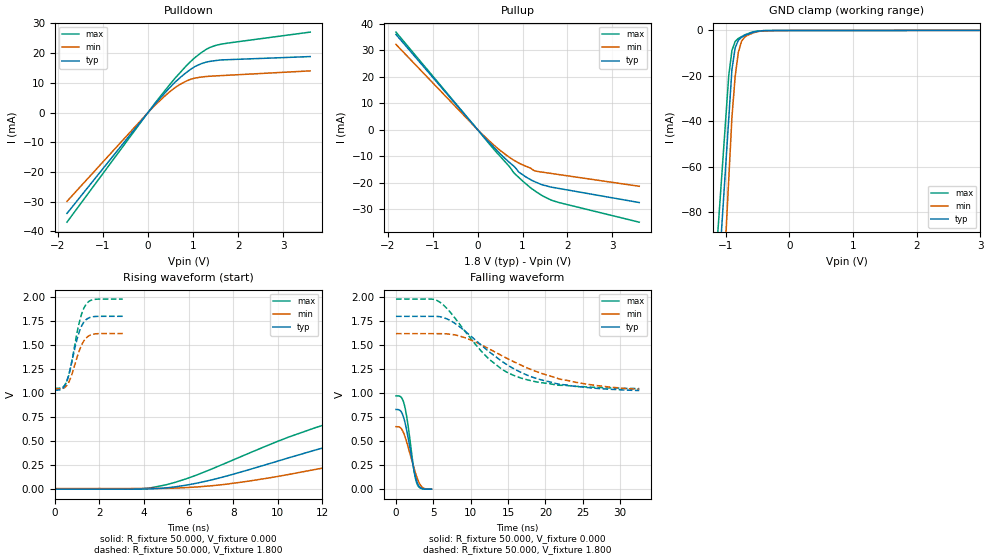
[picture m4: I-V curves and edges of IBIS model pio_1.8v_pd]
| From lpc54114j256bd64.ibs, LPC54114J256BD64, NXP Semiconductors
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[Model]   pio_1.8v_pd
Model_type I/O
Vinl=4.000E-01
Vinh=1.500E+00
Vref=0.000E+00
Rref=1.000E+06
Cref=2.000E-11
Vmeas=9.000E-01
C_comp   9.060E-12   8.700E-12   9.420E-12
[Voltage Range]   1.800E+00   1.620E+00   1.980E+00
[POWER Clamp Reference]   1.800E+00   1.620E+00   1.980E+00
[GND Clamp Reference]   0.000E+00   0.000E+00   0.000E+00
[Pullup Reference]   1.800E+00   1.620E+00   1.980E+00
[Pulldown Reference]   0.000E+00   0.000E+00   0.000E+00
[Temperature Range]   25   105   -40
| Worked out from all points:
|   slope of the pulldown table from 0 to 0.27 V, typ, clamps not added: 55.9 ohm
|   slope of the pullup table from 0 to 0.27 V, typ, clamps not added: 53.5 ohm
|   GND clamp passes 1 mA (typ) near -0.59 V on its own axis
|   rising waveform, R_fixture 50.000, V_fixture 0.000: 20-80 % time 8.49ns typ, 10.2ns min, 6.96ns max; typ from -0.006 V to 0.824 V
|   falling waveform, R_fixture 50.000, V_fixture 0.000: 20-80 % time 1.2ns typ, 1.45ns min, 1.03ns max; typ from 0.83 V to 0 V
|   rising waveform, R_fixture 50.000, V_fixture 1.800: 20-80 % time 492ps typ, 502ps min, 486ps max; typ from 1.03 V to 1.8 V
|   falling waveform, R_fixture 50.000, V_fixture 1.800: 20-80 % time 8.49ns typ, 10.1ns min, 6.71ns max; typ from 1.8 V to 1.03 V
[GND Clamp]
-1.8V     -407.8mA   -530.1mA   -362mA
-950mV    -38.84mA   -65.54mA   -19.87mA
-900mV    -17.14mA   -38.22mA   -8.822mA
-850mV    -7.714mA   -20.45mA   -4.848mA
-800mV    -4.295mA   -9.707mA   -3.501mA
-750mV    -2.992mA   -4.775mA   -2.724mA
-700mV    -2.198mA   -2.883mA   -1.947mA
-550mV    -629.8uA   -893.1uA   -475.4uA
-450mV    -202.6uA   -255.3uA   -151.7uA
3.6V      64.79uA    77.25uA    67.44uA
[Power Clamp]
-1.8V     0A         0A         0A
0V        0A         0A         0A
1.8V      0A         0A         0A
3.6V      0A         0A         0A
[Pullup]
-1.82V    35.96mA    32.21mA    36.85mA
80mV      -1.544mA   -1.344mA   -1.647mA
500mV     -9.045mA   -7.794mA   -9.994mA
700mV     -12.23mA   -10.32mA   -13.77mA
800mV     -13.69mA   -11.44mA   -16.11mA
940mV     -16.27mA   -12.77mA   -18.38mA
1.16V     -18.65mA   -14.36mA   -21.65mA
1.26V     -19.53mA   -15.44mA   -22.89mA
1.44V     -20.77mA   -16.02mA   -24.89mA
1.66V     -21.72mA   -16.55mA   -26.68mA
3.6V      -27.48mA   -21.34mA   -34.89mA
[Pulldown]
-1.8V     -34.01mA   -29.94mA   -36.95mA
0V        0A         0A         0A
380mV     6.716mA    5.665mA    7.485mA
600mV     10.22mA    8.397mA    11.57mA
840mV     13.38mA    10.54mA    15.59mA
1.02V     15.31mA    11.52mA    18.23mA
1.16V     16.32mA    11.92mA    19.92mA
1.38V     17.25mA    12.23mA    21.97mA
1.62V     17.72mA    12.43mA    23.02mA
3.6V      18.85mA    14.03mA    27.1mA
[Rising Waveform]
R_fixture = 50.000
V_fixture = 0.000
V_fixture_min = 0.000
V_fixture_max = 0.000
|  time   V(typ)   V(min)   V(max)
0s        -5.789mV   897uV      -4.844mV
3.7ns     -4.923mV   1.077mV    -2.372mV
4.95ns    6.383mV    2.746mV    37.73mV
7.05ns    91.82mV    30.14mV    206.2mV
11.75ns   407.3mV    203.1mV    641.5mV
13.6ns    519.6mV    285.7mV    761.3mV
15.5ns    613.2mV    364.7mV    841.4mV
20.9ns    764.1mV    537.3mV    935mV
25.8ns    810.2mV    621.3mV    959mV
30.1ns    823.9mV    650.8mV    967.2mV
[Falling Waveform]
R_fixture = 50.000
V_fixture = 0.000
V_fixture_min = 0.000
V_fixture_max = 0.000
|  time   V(typ)   V(min)   V(max)
0s        830.1mV    650.8mV    971.6mV
650ps     811.8mV    635.5mV    960.8mV
900ps     775.2mV    606.4mV    931mV
1.15ns    712.3mV    559.9mV    869.8mV
1.6ns     546.2mV    445.6mV    672.3mV
2.4ns     200.9mV    224.5mV    201.5mV
2.8ns     75.5mV     123.9mV    59.58mV
3.1ns     28.62mV    66.12mV    20.19mV
3.55ns    5.842mV    18.28mV    3.843mV
4.75ns    35.19uV    897uV      149.8uV
[Rising Waveform]
R_fixture = 50.000
V_fixture = 1.800
V_fixture_min = 1.620
V_fixture_max = 1.980
|  time   V(typ)   V(min)   V(max)
0s        1.028V     1.04V      1.048V
350ps     1.047V     1.046V     1.059V
550ps     1.131V     1.081V     1.128V
700ps     1.257V     1.15V      1.256V
1.05ns    1.603V     1.408V     1.686V
1.2ns     1.697V     1.498V     1.821V
1.4ns     1.764V     1.571V     1.924V
1.55ns    1.786V     1.598V     1.958V
1.75ns    1.797V     1.614V     1.975V
3.05ns    1.8V       1.62V      1.98V
[Falling Waveform]
R_fixture = 50.000
V_fixture = 1.800
V_fixture_min = 1.620
V_fixture_max = 1.980
|  time   V(typ)   V(min)   V(max)
0s        1.8V       1.62V      1.98V
4.75ns    1.8V       1.62V      1.98V
5.8ns     1.797V     1.619V     1.952V
8.15ns    1.713V     1.602V     1.756V
12.3ns    1.442V     1.468V     1.366V
14.15ns   1.333V     1.391V     1.25V
16.25ns   1.234V     1.309V     1.17V
21.75ns   1.095V     1.151V     1.083V
26.55ns   1.052V     1.082V     1.061V
32.55ns   1.028V     1.04V      1.048V
[Ramp]
dV/dt_r   4.9781E-01/8.4744E-09   3.9098E-01/1.0185E-08   5.8325E-01/6.9452E-09
dV/dt_f   4.6327E-01/8.4811E-09   3.4800E-01/1.0136E-08   5.5946E-01/6.7072E-09
R_load = 50
